(* Logix 5000 AddOnInstructionDefinition export L_ROTR; software revision 17.00 *)

ADD_ON_INSTRUCTION L_ROTR   (* revision 2.0 20180219, vendor Kenneth A. Fischer *)
// LINT circular right shift (rotation) of the 64-bit argument Inp_A by Inp_B bits
// Revision note:
// Rev2.0: 20180219 - Corrected an error where an Inp_B = 0 results in no output being generated
// Rev1.0: 20170524 - Initial Release
VAR_IN_OUT
   Inp_A : LINT; {required}   // 64-bit Integer to be right circular rotated
END_VAR
VAR_INPUT
   Inp_B : INT; {required}   // Number of Inp_A bit rotations
END_VAR
VAR_IN_OUT
   Out : LINT; {required}   // Result
END_VAR
VAR
   Wrk_InpA : DINT[2];   // Input A as two 32-bit DINTs
   BSR_Cntrl : CONTROL := (LEN := 64);
   Source_Bit : BOOL;
   ONS : BOOL;
END_VAR

ROUTINE Logic   (* ladder *)
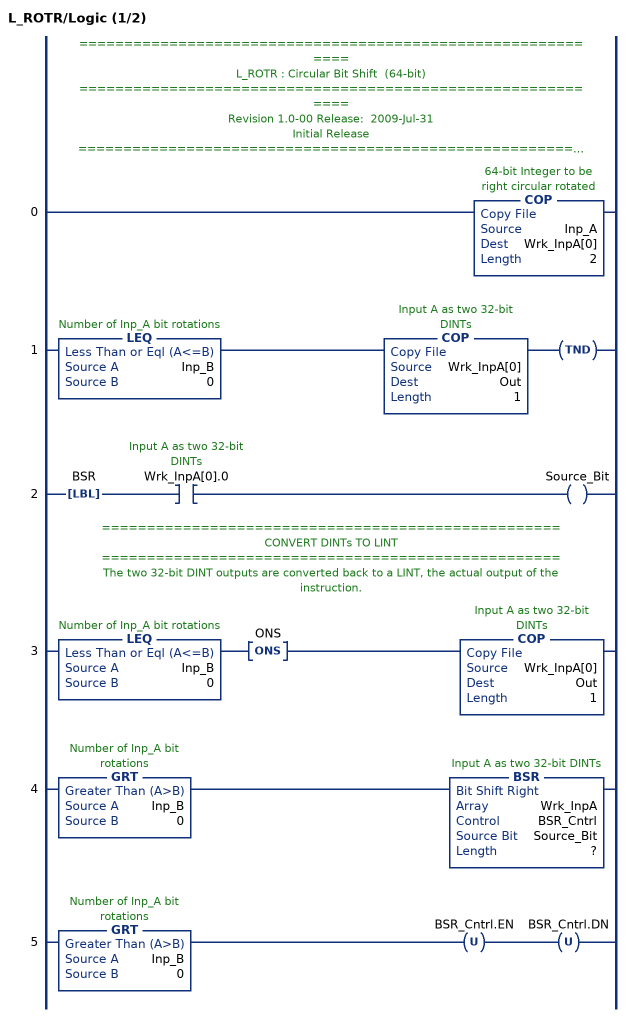
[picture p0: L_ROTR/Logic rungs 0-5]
   // ============================================================
   // L_ROTR : Circular Bit Shift  (64-bit)
   // ============================================================
   // Revision 1.0-00 Release:  2009-Jul-31
   // Initial Release
   // ============================================================
   // Performs a circular right shift rotation of the 64-bit argument Inp_A by the
   // number of bits defined in the 16-bit argument Inp_B.
   // ===================================================
   // CONVERT LINTs TO DINTs
   // ===================================================
   // These COPies take the input LINTs and break them into pairs of DINTs so we can do math on them.
   // Logix V17 has a LINT data type, but math instructions (and AOI Input and Output Parameters) don't support LINT.
   0: COP(Inp_A,Wrk_InpA[0],2);
   1: LEQ(Inp_B,0)COP(Wrk_InpA[0],Out,1)TND();
   2: LBL(BSR)XIC(Wrk_InpA[0].0)OTE(Source_Bit);
   // ===================================================
   // CONVERT DINTs TO LINT
   // ===================================================
   // The two 32-bit DINT outputs are converted back to a LINT, the actual output of the instruction.
   3: LEQ(Inp_B,0)ONS(ONS)COP(Wrk_InpA[0],Out,1);
   4: GRT(Inp_B,0)BSR(Wrk_InpA,BSR_Cntrl,Source_Bit,?);
   5: GRT(Inp_B,0)OTU(BSR_Cntrl.EN)OTU(BSR_Cntrl.DN);
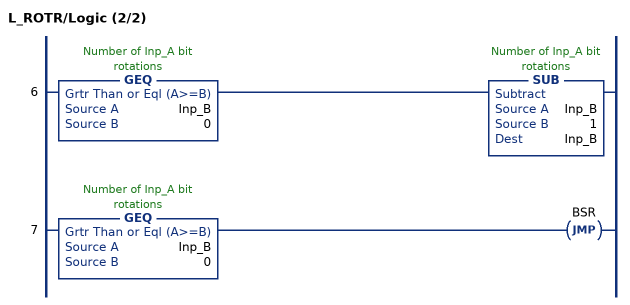
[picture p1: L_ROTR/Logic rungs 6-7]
   6: GEQ(Inp_B,0)SUB(Inp_B,1,Inp_B);
   7: GEQ(Inp_B,0)JMP(BSR);
END_ROUTINE
END_ADD_ON_INSTRUCTION
